| IBIS file stm32g031_041_ufqfpn48.ibs
[IBIS ver] 4.2
[File name] stm32g031_041_ufqfpn48.ibs
[File Rev] rev1.1
[Date]  15-05-2022
[Source] Data Created at STMicroelectronics
[Notes]  File originated from ELDO simulations.
[Disclaimer]  This information is for modeling purpose only and is
   not guaranted. The information is subject to change without
   notice.
[Copyright] Copyright 2022 STMicroelectronics Inc.
|   Component stm32g031_041_ufqfpn48
[Component] stm32g031_041_ufqfpn48
[Manufacturer] STMicroelectronics
[Package]
| variable   typ   min   max
R_pkg   0.0   0.0   0.0
L_pkg   0.0H   0.0H   0.0H
C_pkg   0.0F   0.0F   0.0F
[Pin]   signal_name   model_name  R_pin L_pin C_pin
1 PC13 io8prog2m25m50m120m_sudq_ft
2 PC14-OSC32_IN io8prog2m25m50m120m_sudq_ft
3 PC15-OSC32_OUT io8prog2m25m50m120m_sudq_ft
4 VBAT POWER
5 VREF+ POWER
6 VDDA POWER
7 VSS GND
8 PF0-OSC_IN io6_ft
9 PF1-OSC_OUT io6_ft
10 PF2-NRST io6reset
11 PA0 io6_ft
12 PA1 io6_ft
13 PA2 io6_ft
14 PA3 io6_ft
15 PA4 io6_ft
16 PA5 io6_ft
17 PA6 io6_ft
18 PA7 io6_ft
19 PB0 io6_ft
20 PB1 io6_ft
21 PB2 io6_ft
22 PB10 io6_i2c_ft
23 PB11 io6_i2c_ft
24 PB12 io6_ft
25 PB13 io6_i2c_ft
26 PB14 io6_i2c_ft
27 PB15 io6_ft
28 PA8 io6_ft
29 PA9 io6_i2c_ft
30 PC6 io6_ft
31 PC7 io6_ft
32 PA10 io6_i2c_ft
33 PA11 io6_i2c_ft
34 PA12 io6_i2c_ft
35 PA13 io6_ft
36 PA14-BOOT0 io6_ft
37 PA15 io6_ft
38 PD0 io6_ft
39 PD1 io6_ft
40 PD2 io6_ft
41 PD3 io6_ft
42 PB3 io6_ft
43 PB4 io6_ft
44 PB5 io6_ft
45 PB6 io6_i2c_ft
46 PB7 io6_i2c_ft
47 PB8 io6_i2c_ft
48 PB9 io6_i2c_ft
[Model Selector] io8prog2m25m50m120m_sudq_ft
iols8p_sudq_ft_pd_lv  "IO low speed, PD=40kOhm - 1P8V"
iols8p_sudq_ft_pu_lv  "IO low speed, PU=40kOhm - 1P8V"
iols8p_sudq_ft_lv  "IO low speed - 1P8V"
iols8p_sudq_ft_pd  "IO low speed, PD=40kOhm - 3P3V"
iols8p_sudq_ft_pu  "IO low speed, PU=40kOhm - 3P3V"
iols8p_sudq_ft  "IO low speed - 3P3V"
iofs8p_sudq_ft_pd_lv  "IO full speed, PD=40kOhm - 1P8V"
iofs8p_sudq_ft_pu_lv  "IO full speed, PU=40kOhm - 1P8V"
iofs8p_sudq_ft_lv  "IO full speed - 1P8V"
iofs8p_sudq_ft_pd  "IO full speed, PD=40kOhm - 3P3V"
iofs8p_sudq_ft_pu  "IO full speed, PU=40kOhm - 3P3V"
iofs8p_sudq_ft  "IO full speed - 3P3V"
ioms8p_sudq_ft_pd_lv  "IO medium speed, PD=40kOhm - 1P8V"
ioms8p_sudq_ft_pu_lv  "IO medium speed, PU=40kOhm - 1P8V"
ioms8p_sudq_ft_lv  "IO medium speed - 1P8V"
ioms8p_sudq_ft_pd  "IO medium speed, PD=40kOhm - 3P3V"
ioms8p_sudq_ft_pu  "IO medium speed, PU=40kOhm - 3P3V"
ioms8p_sudq_ft  "IO medium speed - 3P3V"
iohs8p_sudq_ft_pd_lv  "IO high speed, PD=40kOhm - 1P8V"
iohs8p_sudq_ft_pu_lv  "IO high speed, PU=40kOhm - 1P8V"
iohs8p_sudq_ft_lv  "IO high speed - 1P8V"
iohs8p_sudq_ft_pd  "IO high speed, PD=40kOhm - 3P3V"
iohs8p_sudq_ft_pu  "IO high speed, PU=40kOhm - 3P3V"
iohs8p_sudq_ft  "IO high speed - 3P3V"
[Model Selector] io6_ft
io6_ft_1v8_highspeed_pd  "GPIO-1.8V range - high speed - pull down"
io6_ft_1v8_fastspeed_pd  "GPIO-1.8V range - fast speed - pull down"
io6_ft_1v8_mediumspeed_pd  "GPIO-1.8V range - medium speed - pull down"
io6_ft_1v8_lowspeed_pd  "GPIO-1.8V range - low speed - pull down"
io6_ft_1v8_highspeed_pu  "GPIO-1.8V range - high speed - pull up"
io6_ft_1v8_fastspeed_pu  "GPIO-1.8V range - fast speed - pull up"
io6_ft_1v8_mediumspeed_pu  "GPIO-1.8V range - medium speed - pull up"
io6_ft_1v8_lowspeed_pu  "GPIO-1.8V range - low speed - pull up"
io6_ft_1v8_highspeed  "GPIO-1.8V range - high speed"
io6_ft_1v8_fastspeed  "GPIO-1.8V range - fast speed"
io6_ft_1v8_mediumspeed  "GPIO-1.8V range - medium speed"
io6_ft_1v8_lowspeed  "GPIO-1.8V range - low speed"
io6_ft_3v3_highspeed_pd  "GPIO-3.3V range - high speed - pull down"
io6_ft_3v3_fastspeed_pd  "GPIO-3.3V range - fast speed - pull down"
io6_ft_3v3_mediumspeed_pd  "GPIO-3.3V range - medium speed - pull down"
io6_ft_3v3_lowspeed_pd  "GPIO-3.3V range - low speed - pull down"
io6_ft_3v3_highspeed_pu  "GPIO-3.3V range - high speed - pull up"
io6_ft_3v3_fastspeed_pu  "GPIO-3.3V range - fast speed - pull up"
io6_ft_3v3_mediumspeed_pu  "GPIO-3.3V range - medium speed - pull up"
io6_ft_3v3_lowspeed_pu  "GPIO-3.3V range - low speed - pull up"
io6_ft_3v3_highspeed  "GPIO-3.3V range - high speed"
io6_ft_3v3_fastspeed  "GPIO-3.3V range - fast speed"
io6_ft_3v3_mediumspeed  "GPIO-3.3V range - medium speed"
io6_ft_3v3_lowspeed  "GPIO-3.3V range - low speed"
[Model Selector] io6_i2c_ft
io6_ft_1v8_highspeed_pd  "GPIO-1.8V range - high speed - pull down"
io6_ft_1v8_fastspeed_pd  "GPIO-1.8V range - fast speed - pull down"
io6_ft_1v8_mediumspeed_pd  "GPIO-1.8V range - medium speed - pull down"
io6_ft_1v8_lowspeed_pd  "GPIO-1.8V range - low speed - pull down"
io6_ft_1v8_highspeed_pu  "GPIO-1.8V range - high speed - pull up"
io6_ft_1v8_fastspeed_pu  "GPIO-1.8V range - fast speed - pull up"
io6_ft_1v8_mediumspeed_pu  "GPIO-1.8V range - medium speed - pull up"
io6_ft_1v8_lowspeed_pu  "GPIO-1.8V range - low speed - pull up"
io6_ft_1v8_highspeed  "GPIO-1.8V range - high speed"
io6_ft_1v8_fastspeed  "GPIO-1.8V range - fast speed"
io6_ft_1v8_mediumspeed  "GPIO-1.8V range - medium speed"
io6_ft_1v8_lowspeed  "GPIO-1.8V range - low speed"
io6_ft_3v3_highspeed_pd  "GPIO-3.3V range - high speed - pull down"
io6_ft_3v3_fastspeed_pd  "GPIO-3.3V range - fast speed - pull down"
io6_ft_3v3_mediumspeed_pd  "GPIO-3.3V range - medium speed - pull down"
io6_ft_3v3_lowspeed_pd  "GPIO-3.3V range - low speed - pull down"
io6_ft_3v3_highspeed_pu  "GPIO-3.3V range - high speed - pull up"
io6_ft_3v3_fastspeed_pu  "GPIO-3.3V range - fast speed - pull up"
io6_ft_3v3_mediumspeed_pu  "GPIO-3.3V range - medium speed - pull up"
io6_ft_3v3_lowspeed_pu  "GPIO-3.3V range - low speed - pull up"
io6_ft_3v3_highspeed  "GPIO-3.3V range - high speed"
io6_ft_3v3_fastspeed  "GPIO-3.3V range - fast speed"
io6_ft_3v3_mediumspeed  "GPIO-3.3V range - medium speed"
io6_ft_3v3_lowspeed  "GPIO-3.3V range - low speed"
io6_ft_1v8_highi2c_pd   "GPIO-1.8V range - high   speed i2c mode - pd"
io6_ft_1v8_fasti2c_pd   "GPIO-1.8V range - fast   speed i2c mode - pd"
io6_ft_1v8_mediumi2c_pd  "GPIO-1.8V range - medium speed i2c mode - pd"
io6_ft_1v8_lowi2c_pd   "GPIO-1.8V range - low   speed i2c mode - pd"
io6_ft_1v8_highi2c_pu   "GPIO-1.8V range - high   speed i2c mode - pu"
io6_ft_1v8_fasti2c_pu   "GPIO-1.8V range - fast   speed i2c mode - pu"
io6_ft_1v8_mediumi2c_pu  "GPIO-1.8V range - medium speed i2c mode - pu"
io6_ft_1v8_lowi2c_pu   "GPIO-1.8V range - low   speed i2c mode - pu"
io6_ft_1v8_highi2c   "GPIO-1.8V range - high   speed i2c mode"
io6_ft_1v8_fasti2c   "GPIO-1.8V range - fast   speed i2c mode"
io6_ft_1v8_mediumi2c   "GPIO-1.8V range - medium speed i2c mode"
io6_ft_1v8_lowi2c   "GPIO-1.8V range - low   speed i2c mode"
io6_ft_3v3_highi2c_pd   "GPIO-3.3V range - high   speed i2c mode - pd"
io6_ft_3v3_fasti2c_pd   "GPIO-3.3V range - fast   speed i2c mode - pd"
io6_ft_3v3_mediumi2c_pd  "GPIO-3.3V range - medium speed i2c mode - pd"
io6_ft_3v3_lowi2c_pd   "GPIO-3.3V range - low   speed i2c mode - pd"
io6_ft_3v3_highi2c_pu   "GPIO-3.3V range - high   speed i2c mode - pu"
io6_ft_3v3_fasti2c_pu   "GPIO-3.3V range - fast   speed i2c mode - pu"
io6_ft_3v3_mediumi2c_pu  "GPIO-3.3V range - medium speed i2c mode - pu"
io6_ft_3v3_lowi2c_pu   "GPIO-3.3V range - low   speed i2c mode - pu"
io6_ft_3v3_highi2c   "GPIO-3.3V range - high   speed i2c mode"
io6_ft_3v3_fasti2c   "GPIO-3.3V range - fast   speed i2c mode"
io6_ft_3v3_mediumi2c   "GPIO-3.3V range - medium speed i2c mode"
io6_ft_3v3_lowi2c   "GPIO-3.3V range - low   speed i2c mode"
io6_i2c_ft_1v8_pd  "GPIO-1.8V I2C fm+ - pd"
io6_i2c_ft_3v3_pd  "GPIO-3.3V I2C fm+ - pd"
io6_i2c_ft_1v8_pu  "GPIO-1.8V I2C fm+ - pu"
io6_i2c_ft_3v3_pu  "GPIO-3.3V I2C fm+ - pu"
io6_i2c_ft_1v8   "GPIO-1.8V I2C fm+"
io6_i2c_ft_3v3   "GPIO-3.3V I2C fm+"
[Model Selector] io6reset
io6_ft_1v8_highspeed_pd  "GPIO-1.8V range - high speed - pull down"
io6_ft_1v8_fastspeed_pd  "GPIO-1.8V range - fast speed - pull down"
io6_ft_1v8_mediumspeed_pd  "GPIO-1.8V range - medium speed - pull down"
io6_ft_1v8_lowspeed_pd  "GPIO-1.8V range - low speed - pull down"
io6_ft_1v8_highspeed_pu  "GPIO-1.8V range - high speed - pull up"
io6_ft_1v8_fastspeed_pu  "GPIO-1.8V range - fast speed - pull up"
io6_ft_1v8_mediumspeed_pu  "GPIO-1.8V range - medium speed - pull up"
io6_ft_1v8_lowspeed_pu  "GPIO-1.8V range - low speed - pull up"
io6_ft_1v8_highspeed  "GPIO-1.8V range - high speed"
io6_ft_1v8_fastspeed  "GPIO-1.8V range - fast speed"
io6_ft_1v8_mediumspeed  "GPIO-1.8V range - medium speed"
io6_ft_1v8_lowspeed  "GPIO-1.8V range - low speed"
io6_ft_3v3_highspeed_pd  "GPIO-3.3V range - high speed - pull down"
io6_ft_3v3_fastspeed_pd  "GPIO-3.3V range - fast speed - pull down"
io6_ft_3v3_mediumspeed_pd  "GPIO-3.3V range - medium speed - pull down"
io6_ft_3v3_lowspeed_pd  "GPIO-3.3V range - low speed - pull down"
io6_ft_3v3_highspeed_pu  "GPIO-3.3V range - high speed - pull up"
io6_ft_3v3_fastspeed_pu  "GPIO-3.3V range - fast speed - pull up"
io6_ft_3v3_mediumspeed_pu  "GPIO-3.3V range - medium speed - pull up"
io6_ft_3v3_lowspeed_pu  "GPIO-3.3V range - low speed - pull up"
io6_ft_3v3_highspeed  "GPIO-3.3V range - high speed"
io6_ft_3v3_fastspeed  "GPIO-3.3V range - fast speed"
io6_ft_3v3_mediumspeed  "GPIO-3.3V range - medium speed"
io6_ft_3v3_lowspeed  "GPIO-3.3V range - low speed"
ioreset_1v2_pu  "RESET 1.2V range with PU"
ioreset_1v2  "RESET 1.2V range"
ioreset_1v8_pu  "RESET 1.8V range with PU"
ioreset_1v8  "RESET 1.8V range"
ioreset_3v3_pu  "RESET 3.3V range with PU"
ioreset_3v3  "RESET 3.3V range"
| Models and submodels in the file (84): iols8p_sudq_ft_pd_lv (I/O), iols8p_sudq_ft_pu_lv (I/O), iols8p_sudq_ft_lv (I/O), iols8p_sudq_ft_pd (I/O), iols8p_sudq_ft_pu (I/O), iols8p_sudq_ft (I/O), iofs8p_sudq_ft_pd_lv (I/O), iofs8p_sudq_ft_pu_lv (I/O), iofs8p_sudq_ft_lv (I/O), iofs8p_sudq_ft_pd (I/O), iofs8p_sudq_ft_pu (I/O), iofs8p_sudq_ft (I/O), ioms8p_sudq_ft_pd_lv (I/O), ioms8p_sudq_ft_pu_lv (I/O), ioms8p_sudq_ft_lv (I/O), ioms8p_sudq_ft_pd (I/O), ioms8p_sudq_ft_pu (I/O), ioms8p_sudq_ft (I/O), iohs8p_sudq_ft_pd_lv (I/O), iohs8p_sudq_ft_pu_lv (I/O), iohs8p_sudq_ft_lv (I/O), iohs8p_sudq_ft_pd (I/O), iohs8p_sudq_ft_pu (I/O), iohs8p_sudq_ft (I/O), io6_ft_1v8_highspeed_pd (I/O), io6_ft_1v8_fastspeed_pd (I/O), io6_ft_1v8_mediumspeed_pd (I/O), io6_ft_1v8_lowspeed_pd (I/O), io6_ft_1v8_highspeed_pu (I/O), io6_ft_1v8_fastspeed_pu (I/O), io6_ft_1v8_mediumspeed_pu (I/O), io6_ft_1v8_lowspeed_pu (I/O), io6_ft_1v8_highspeed (I/O), io6_ft_1v8_fastspeed (I/O), io6_ft_1v8_mediumspeed (I/O), io6_ft_1v8_lowspeed (I/O), io6_ft_3v3_highspeed_pd (I/O), io6_ft_3v3_fastspeed_pd (I/O), io6_ft_3v3_mediumspeed_pd (I/O), io6_ft_3v3_lowspeed_pd (I/O), io6_ft_3v3_highspeed_pu (I/O), io6_ft_3v3_fastspeed_pu (I/O), io6_ft_3v3_mediumspeed_pu (I/O), io6_ft_3v3_lowspeed_pu (I/O), io6_ft_3v3_highspeed (I/O), io6_ft_3v3_fastspeed (I/O), io6_ft_3v3_mediumspeed (I/O), io6_ft_3v3_lowspeed (I/O), io6_i2c_ft_1v8_pd (I/O_open_drain), io6_i2c_ft_3v3_pd (I/O_open_drain), io6_i2c_ft_1v8_pu (I/O_open_drain), io6_i2c_ft_3v3_pu (I/O_open_drain), io6_i2c_ft_1v8 (I/O_open_drain), io6_i2c_ft_3v3 (I/O_open_drain), io6_ft_1v8_highi2c_pd (I/O_open_drain), io6_ft_1v8_fasti2c_pd (I/O_open_drain), io6_ft_1v8_mediumi2c_pd (I/O_open_drain), io6_ft_1v8_lowi2c_pd (I/O_open_drain), io6_ft_1v8_highi2c_pu (I/O_open_drain), io6_ft_1v8_fasti2c_pu (I/O_open_drain), io6_ft_1v8_mediumi2c_pu (I/O_open_drain), io6_ft_1v8_lowi2c_pu (I/O_open_drain), io6_ft_1v8_highi2c (I/O_open_drain), io6_ft_1v8_fasti2c (I/O_open_drain), io6_ft_1v8_mediumi2c (I/O_open_drain), io6_ft_1v8_lowi2c (I/O_open_drain), io6_ft_3v3_highi2c_pd (I/O_open_drain), io6_ft_3v3_fasti2c_pd (I/O_open_drain), io6_ft_3v3_mediumi2c_pd (I/O_open_drain), io6_ft_3v3_lowi2c_pd (I/O_open_drain), io6_ft_3v3_highi2c_pu (I/O_open_drain), io6_ft_3v3_fasti2c_pu (I/O_open_drain), io6_ft_3v3_mediumi2c_pu (I/O_open_drain), io6_ft_3v3_lowi2c_pu (I/O_open_drain), io6_ft_3v3_highi2c (I/O_open_drain), io6_ft_3v3_fasti2c (I/O_open_drain), io6_ft_3v3_mediumi2c (I/O_open_drain), io6_ft_3v3_lowi2c (I/O_open_drain), ioreset_1v2_pu (I/O_open_drain), ioreset_1v2 (I/O_open_drain)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
